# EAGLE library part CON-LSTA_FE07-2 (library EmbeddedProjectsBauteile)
FEMALE HEADER 2x7pins
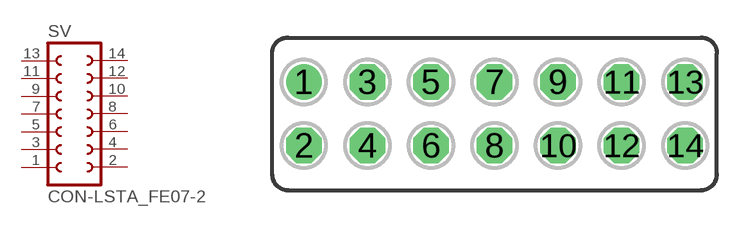
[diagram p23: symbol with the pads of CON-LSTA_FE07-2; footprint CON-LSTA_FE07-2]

Designator prefix SV

## CON-LSTA_FE07-2  [CON-LSTA_FE07-2]
1  1  pas
2  2  pas
3  3  pas
4  4  pas
5  5  pas
6  6  pas
7  7  pas
8  8  pas
9  9  pas
10  10  pas
11  11  pas
12  12  pas
13  13  pas
14  14  pas

## Footprint CON-LSTA_FE07-2 (pad centres in mm)
drill 0.914: 1 -7.62,1.27
drill 0.914 octagon: 2 -7.62,-1.27; 3 -5.08,1.27; 4 -5.08,-1.27; 5 -2.54,1.27; 6 -2.54,-1.27; 7 0,1.27; 8 0,-1.27; 9 2.54,1.27; 10 2.54,-1.27; 11 5.08,1.27; 12 5.08,-1.27; 13 7.62,1.27; 14 7.62,-1.27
